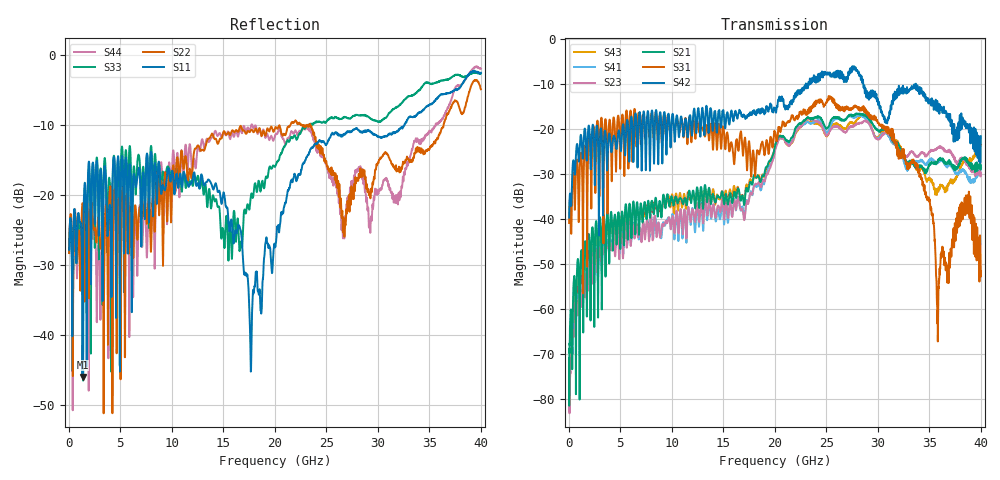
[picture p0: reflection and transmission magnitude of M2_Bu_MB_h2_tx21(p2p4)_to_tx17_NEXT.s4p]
! S11 = S11
! S12 = S12
! S13 = S13
! S14 = S14
! S21 = S21
! S22 = S22
! S23 = S23
! S24 = S24
! S31 = S31
! S32 = S32
! S33 = S33
! S34 = S34
! S41 = S41
! S42 = S42
! S43 = S43
! S44 = S44
! FILE: \\englab.brocade.com\shares\Groups\SIT\Work\Shaohua\IEEE_channels\M2_Bu_MB_h2_tx21(p2p4)_to_tx17_NEXT.s4p
!$DUT_CFG_DESC: Default 4-Port Configuration
!$NUMBER_PORTS: 4
!$DIFF_PORT_MAP: 1|2P|2|2P|0|UC|0|UC|
!$PORT_MAP: PNA 1|1|<<<<<<|TS 2|2|>>>>>>|PNA 2|3|<<<<<<|TS 4|4|>>>>>>|
# MHz S RI R 50.00
! FREQ  S11  S12  S13  S14
!  S21  S22  S23  S24
!  S31  S32  S33  S34
!  S41  S42  S43  S44
!  REAL  IMAG  REAL  IMAG  REAL  IMAG  REAL  IMAG
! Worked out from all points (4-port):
!   3996 points, 50 MHz to 40 GHz, reference 50 ohm
!   strongest paths, dB at 50 MHz, 10.04 GHz, 20.03 GHz, 30.02 GHz, 40 GHz:
!     S42: -39.7, -17.1, -15.7, -13.8, -21.7
!     S31: -40.9, -18.3, -20.7, -18.7, -51.6
!     S21: -71.0, -35.4, -23.7, -20.3, -28.1
!     S23: -77.7, -39.9, -24.8, -22.4, -29.8
!     S41: -75.7, -39.2, -24.5, -22.1, -28.7
!     S43: -75.9, -34.6, -23.8, -21.9, -23.5
!   lowest |S11| = -46.0 dB at 1.35 GHz (marker M1), VSWR 1.01, Z = 49.7 + j0.376 ohm
!   |S11| at or under -10 dB: start of sweep to 32.57 GHz
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50  0.0239 -0.033  -7.86e-05 0.000129  0.00514 0.00774  -2.89e-05 0.000107
    -0.000256 0.000118  0.024 -0.0302  9.68e-05 8.62e-05  0.00595 0.00825
    0.00495 0.00748  6.63e-05 2.89e-05  0.0246 -0.0302  3.03e-05 0.000343
    -0.000132 -9.8e-05  0.00615 0.00826  -0.000129 9.43e-05  0.0234 -0.0309
1350  -0.00332 0.00379  0.00231 0.00145  0.0178 -0.00352  0.000207 0.00167
      0.0023 0.00145  -0.086 -0.0158  -0.00021 0.00194  0.00353 -0.0482
      0.0178 -0.0035  -0.000223 0.00192  0.00827 0.0325  0.000158 0.00278
      0.00021 0.00174  0.00361 -0.0482  0.000157 0.00277  -0.079 -0.0179
17680  0.00548 -0.000497  0.0163 -0.0184  -0.034 -0.000625  0.011 -0.0155
       0.0176 -0.0187  0.069 -0.2811  0.0084 -0.0176  -0.0163 -0.1398
       -0.0337 -0.000587  0.00752 -0.0168  -0.0118 0.0968  0.0152 -0.0197
       0.0122 -0.0161  -0.016 -0.1424  0.0173 -0.0208  0.0719 -0.2976
25380  0.1457 0.2123  -0.0982 0.0469  0.1787 0.1624  -0.0884 0.0207
       -0.101 0.0611  -0.12 -0.0961  -0.0754 0.0601  -0.3294 0.1482
       0.1707 0.1532  -0.0714 0.0469  0.1516 0.3172  -0.0739 0.0367
       -0.0993 0.0374  -0.3483 0.1719  -0.0817 0.0541  -0.128 -0.0497
33600  0.2731 0.2398  0.0339 0.018  -0.00624 -0.0512  0.0234 0.0371
       0.0358 0.0112  0.1974 -0.00227  0.0396 0.0318  -0.1363 0.2549
       -0.00306 -0.0418  0.0258 0.0324  0.2681 0.4512  0.0316 0.00922
       0.0296 0.032  -0.1346 0.2611  0.039 0.00298  0.1758 0.1695
35820  0.3867 0.3105  0.0297 0.023  3.24e-05 -0.000774  0.0271 0.0261
       0.0368 0.0251  0.2425 0.0659  0.05 0.0362  -0.063 0.1478
       7.61e-05 -0.000425  0.0341 0.0319  0.4305 0.4706  0.0128 0.00946
       0.0301 0.0303  -0.0726 0.1385  0.0177 0.0116  0.2531 0.1972
40000  0.7107 0.2263  0.0208 0.0283  0.00478 -0.000462  0.00833 0.0189
       0.0376 0.0117  0.5617 -0.0892  0.0322 0.00317  -0.0475 -0.0181
       0.00262 0.000118  0.00959 0.0122  0.6367 0.3735  0.0139 0.0134
       0.0242 0.0278  -0.0638 -0.0523  0.0631 0.0217  0.7973 0.0432
